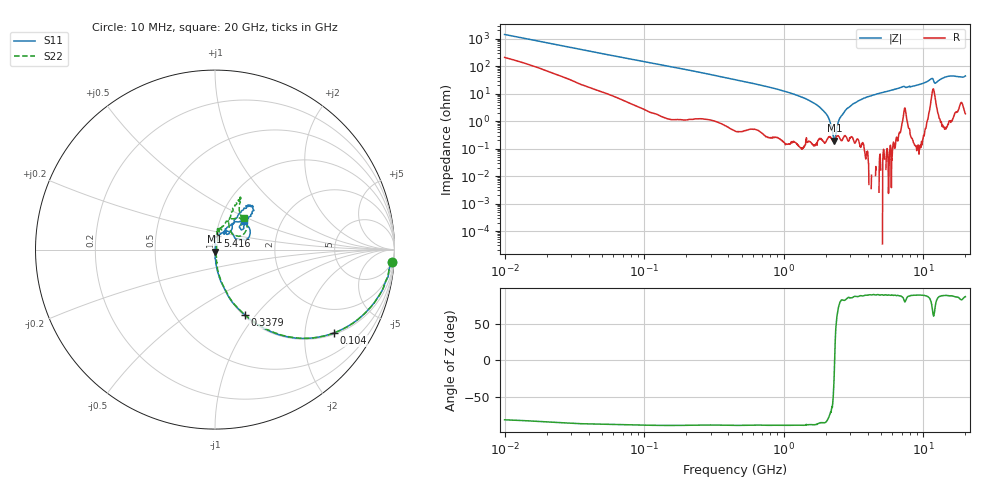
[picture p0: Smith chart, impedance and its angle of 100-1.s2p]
!Keysight Technologies,P5008B,MY61100088,A.16.20.02
!Date: Monday, May 27, 2024 17:05:25
!Correction: S11(C* 2-Port  )
!S21(C* 2-Port  )
!S12(C* 2-Port  )
!S22(C* 2-Port  )
!S2P File: Measurements: S11, S21, S12, S22:Log Frequency Sweep
# Hz S  dB  R 50
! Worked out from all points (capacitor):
!   1601 points, 10 MHz to 20 GHz, reference 50 ohm
!   read as one part in series: C = 11.3 pF near 10.39 MHz
!   lowest |Z| = 196 mohm at 2.303 GHz (marker M1)
!   series resonance near 2.312 GHz, so ESL is about 420 pH
!   S11 on the Smith chart (normalised r, x): 10 MHz: 4, -29; 104 MHz: 1.05, -2.83; 337.9 MHz: 1.01, -0.88; 5.416 GHz: 1.02, +0.15; 20 GHz: 1.30, +0.44
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1e7  -0.09 -3.9  -23.23 77.7  -23.24 77.7  -0.12 -3.9
3.555162e7  -0.37 -13.7  -12.44 73.2  -12.45 73.2  -0.37 -13.8
1.040231e8  -1.83 -34.9  -4.86 54.1  -4.87 54.1  -1.82 -34.9
1.263918e8  -2.43 -40.1  -3.84 49.1  -3.85 49.1  -2.42 -40.1
3.37901e8  -7.99 -65.6  -0.82 23.3  -0.83 23.3  -7.99 -65.4
4.472136e8  -10.14 -71.6  -0.48 17.9  -0.49 17.9  -10.14 -71.3
9.119826e8  -16.73 -81.7  -0.11 7.8  -0.12 7.9  -16.75 -80.7
1.589917e9  -25.02 -87.8  -0.01 2.4  -0.02 2.4  -24.80 -82.6
2.025791e9  -31.22 -88.8  -0.00 0.4  -0.01 0.4  -30.53 -76.2
2.30303e9  -38.23 -89.1  0.00 -0.7  -0.01 -0.7  -36.27 -63.8
2.568928e9  -55.25 55.3  0.00 -1.7  -0.01 -1.6  -43.40 2.1
2.798263e9  -38.69 77.1  0.00 -2.4  -0.01 -2.4  -36.86 51.3
3.136201e9  -32.43 85.1  0.00 -3.5  -0.01 -3.5  -31.15 68.7
3.846973e9  -27.09 93.8  0.00 -5.5  -0.01 -5.5  -25.83 73.1
5.415836e9  -22.51 79.6  -0.01 -9.3  -0.02 -9.3  -22.48 78.7
5.652411e9  -21.74 78.3  -0.01 -9.9  -0.03 -9.9  -21.78 80.3
7.100103e9  -18.29 58.9  -0.10 -13.7  -0.12 -13.7  -18.60 80.1
9.264046e9  -18.93 62.5  -0.03 -18.0  -0.04 -18.0  -18.76 77.8
1.13636e10  -13.12 44.8  -0.66 -25.7  -0.67 -25.7  -13.11 53.4
1.237806e10  -17.21 49.3  -0.35 -20.9  -0.36 -20.9  -17.03 54.6
1.518335e10  -10.17 50.9  -0.45 -30.3  -0.46 -30.3  -10.06 63.4
2e10  -12.82 45.1  -0.34 -38.3  -0.35 -38.4  -12.42 46.8
